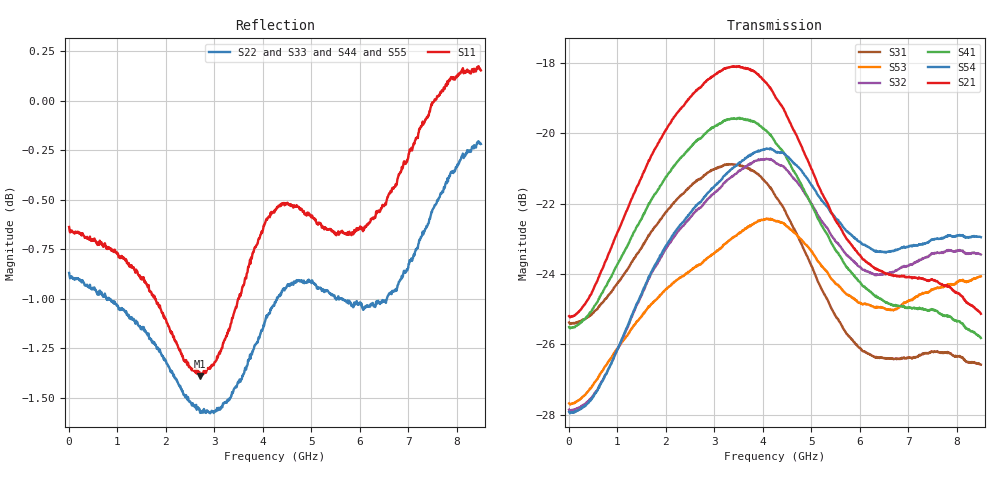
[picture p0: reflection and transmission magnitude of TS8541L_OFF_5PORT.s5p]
! Created with skrf (http://scikit-rf.org).
# Hz S RI R 50.0
!freq ReS11 ImS11 ReS12 ImS12 ReS13 ImS13
! ReS14 ImS14 ReS15 ImS15
! ReS21 ImS21 ReS22 ImS22 ReS23 ImS23
! ReS24 ImS24 ReS25 ImS25
! ReS31 ImS31 ReS32 ImS32 ReS33 ImS33
! ReS34 ImS34 ReS35 ImS35
! ReS41 ImS41 ReS42 ImS42 ReS43 ImS43
! ReS44 ImS44 ReS45 ImS45
! ReS51 ImS51 ReS52 ImS52 ReS53 ImS53
! ReS54 ImS54 ReS55 ImS55
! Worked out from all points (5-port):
!   1601 points, 10 MHz to 8.5 GHz, reference 50 ohm
!   strongest paths, dB at 10 MHz, 2.132 GHz, 4.255 GHz, 6.378 GHz, 8.5 GHz:
!     S21: -25.2, -19.6, -18.9, -23.9, -25.1
!     S54: -27.9, -22.9, -20.5, -23.4, -23.0
!     S41: -25.5, -21.0, -20.2, -24.7, -25.8
!     S32: -27.9, -23.0, -20.8, -24.0, -23.4
!     S53: -27.7, -24.3, -22.5, -24.9, -24.1
!     S31: -25.4, -22.0, -21.8, -26.4, -26.6
!   lowest |S11| = -1.4 dB at 2.711 GHz (marker M1), VSWR 12.52, Z = 6.56 + j39.9 ohm
!   |S11| at or under -10 dB: nowhere
